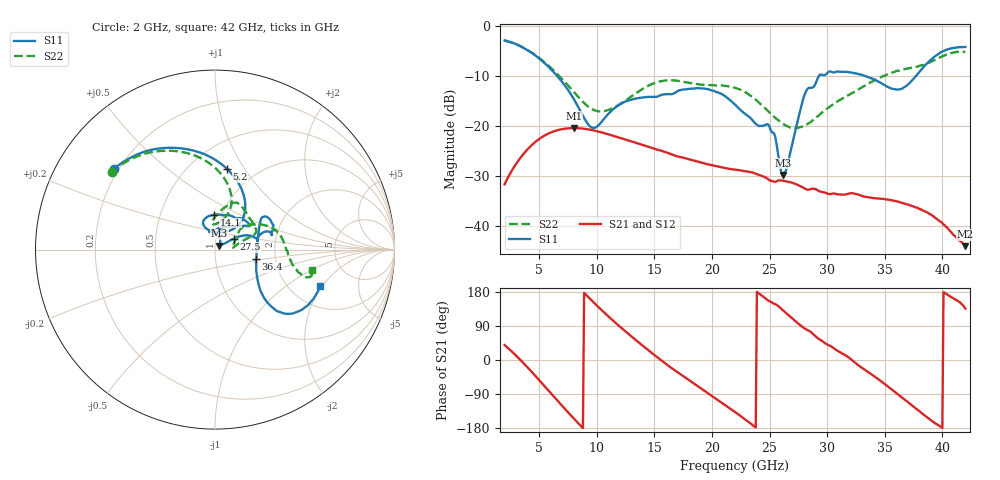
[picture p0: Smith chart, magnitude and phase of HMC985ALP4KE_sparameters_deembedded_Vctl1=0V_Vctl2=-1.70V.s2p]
!s2p File: Measurements: S11, S21, S12, S22
# GHz S dB R 50.0
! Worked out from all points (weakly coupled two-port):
!   401 points, 2 GHz to 42 GHz, reference 50 ohm
!   highest |S21| = -20.36 dB at 8 GHz (marker M1); lowest = -44.0 dB at 42 GHz (marker M2)
!   lowest |S11| = -29.8 dB at 26.2 GHz (marker M3), VSWR 1.07, Z = 52.4 + j2.34 ohm
!   |S11| at or under -10 dB: 6.584 GHz to 29.27 GHz (22.68 GHz wide, 127 % of centre); 33.36 GHz to 37.69 GHz (4.338 GHz wide, 12.2 % of centre)
!   |S22| runs from -20.4 to -2.8 dB; largest |S21 - S12| = 0.00015
!   S11 on the Smith chart (normalised r, x): 2 GHz: 0.18, +0.34; 5.2 GHz: 0.74, +0.84; 14.1 GHz: 0.92, +0.37; 27.5 GHz: 1.22, +0.15; 36.4 GHz: 1.58, -0.18; 42 GHz: 2.90, -1.91
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2  -2.85 141.3  -31.61 39.5  -31.61 39.5  -2.85 143.0
3.5  -4.15 113.8  -25.95 -3.9  -25.95 -3.9  -4.16 117.3
5.2  -6.83 81.7  -22.24 -59.9  -22.24 -59.9  -6.70 90.9
8  -14.54 46.5  -20.36 -154.2  -20.38 -154.3  -13.11 69.8
8.7  -17.50 52.1  -20.45 -176.6  -20.46 -176.6  -14.90 73.7
9.8  -20.33 87.5  -20.87 149.8  -20.88 149.8  -16.81 86.5
12  -15.63 113.6  -22.32 88.2  -22.32 88.2  -15.60 93.6
14.1  -14.22 91.1  -23.82 35.0  -23.83 35.0  -12.36 77.1
15.4  -13.94 73.0  -24.78 4.1  -24.78 4.1  -11.08 69.0
19.4  -12.52 34.4  -27.47 -82.4  -27.48 -82.4  -11.74 38.6
22  -15.66 52.3  -28.68 -137.1  -28.69 -137.2  -12.31 21.8
25  -20.12 98.2  -30.81 154.9  -30.82 154.9  -17.29 14.5
26.2  -29.77 43.3  -30.91 129.9  -30.91 130.0  -19.57 7.3
27.5  -18.37 30.0  -31.80 95.8  -31.81 95.8  -20.28 7.0
28.1  -13.34 20.8  -32.51 82.1  -32.53 82.2  -19.81 12.3
28.7  -12.30 12.9  -32.50 70.8  -32.51 70.8  -18.91 19.0
31  -9.07 23.3  -33.63 22.7  -33.65 22.6  -14.87 38.8
33.3  -9.95 34.3  -34.12 -26.3  -34.12 -26.3  -11.87 33.1
35.4  -12.27 12.2  -34.72 -72.9  -34.73 -72.9  -9.50 21.5
36.4  -12.57 -12.9  -35.25 -96.8  -35.25 -96.8  -8.73 14.7
39.5  -5.81 -43.3  -38.48 -169.1  -38.48 -169.3  -6.53 -14.1
42  -4.14 -19.0  -43.99 135.7  -44.01 135.2  -5.13 -12.0
